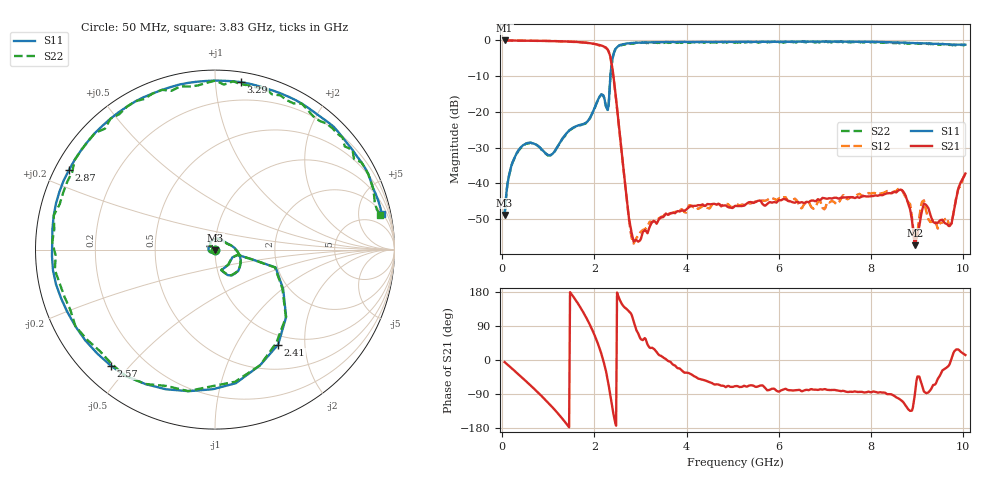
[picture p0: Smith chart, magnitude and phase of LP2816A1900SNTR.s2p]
!	AVX	THIN	FILM	OPERATION
!	LP2816S	High	Performance	Low	Pass	Filters
!	P/N	LP2816A1900SNTR
!	Created	28	January	2020
!Instrument:	"HEWLETT PACKARD,8720ES,US39172150,7.62 "
#	MHz	S	dB	R	50
!	Frq	S11(dB)	S11(deg)	S21(dB)	S21(deg)	S12(dB)	S12(deg)	S22(dB)	S22(deg)
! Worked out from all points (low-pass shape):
!   501 points, 50 MHz to 10.05 GHz, reference 50 ohm
!   highest |S21| = 0.00 dB at 50 MHz (marker M1); lowest = -57.4 dB at 8.95 GHz (marker M2)
!   |S21| within 3 dB of the highest: start of sweep to 2.305 GHz
!   lowest |S11| = -48.9 dB at 50 MHz (marker M3), VSWR 1.01, Z = 50.2 - j0.319 ohm
!   |S11| at or under -10 dB: start of sweep to 2.346 GHz
!   |S22| runs from -48.9 to -0.3 dB; largest |S21 - S12| = 0.033
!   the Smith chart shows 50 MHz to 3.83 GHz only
!   S11 on the Smith chart (normalised r, x): 50 MHz: 1.00, -0.01; 2.41 GHz: 0.85, -1.51; 2.57 GHz: 0.08, -0.44; 2.87 GHz: 0.04, +0.25; 3.29 GHz: 0.07, +1.16; 3.83 GHz: 2.21, +9.03
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50  -48.90 -62.3  0.00 -5.5  0.00 -5.7  -48.90 -62.3
370  -30.42 -150.9  -0.05 -40.1  -0.06 -40.0  -30.62 -151.1
910  -31.24 133.6  -0.14 -102.2  -0.11 -102.1  -31.24 133.4
1390  -26.09 118.0  -0.29 -168.1  -0.30 -168.4  -26.09 117.8
1730  -23.53 49.4  -0.53 131.5  -0.56 131.4  -23.53 49.4
1970  -19.88 9.2  -0.90 74.6  -0.95 74.1  -20.08 9.2
2170  -15.21 -50.0  -1.51 7.8  -1.62 7.2  -15.31 -50.0
2310  -17.63 -13.1  -3.14 -67.8  -3.25 -69.4  -17.83 -13.2
2410  -3.94 -56.4  -9.71 -141.0  -10.25 -140.6  -4.14 -56.5
2570  -1.22 -131.9  -28.46 153.7  -28.96 154.9  -1.32 -131.9
2870  -0.66 151.4  -56.16 93.6  -56.38 94.2  -0.86 151.4
3290  -0.50 81.2  -50.62 29.3  -50.51 27.8  -0.60 81.2
3390  -0.50 67.2  -50.33 14.5  -49.93 18.7  -0.60 67.0
3830  -0.44 11.9  -47.87 -22.1  -47.67 -24.5  -0.54 11.8
4490  -0.41 -60.6  -45.91 -58.3  -47.10 -53.3  -0.61 -60.7
5050  -0.43 -116.3  -46.35 -69.1  -46.07 -66.8  -0.63 -116.5
5870  -0.38 170.6  -45.38 -75.7  -44.24 -76.9  -0.38 170.5
6730  -0.32 103.5  -44.86 -77.5  -46.94 -86.7  -0.42 103.4
8390  -0.48 -24.3  -42.79 -90.0  -42.19 -88.9  -0.48 -24.5
8950  -0.76 -73.5  -57.38 -94.0  -57.65 -108.2  -0.76 -73.7
9710  -1.07 -147.4  -51.98 -10.2  -51.73 -13.7  -1.27 -147.5
10050  -1.19 177.6  -37.29 13.1  -37.46 6.7  -1.39 177.6
